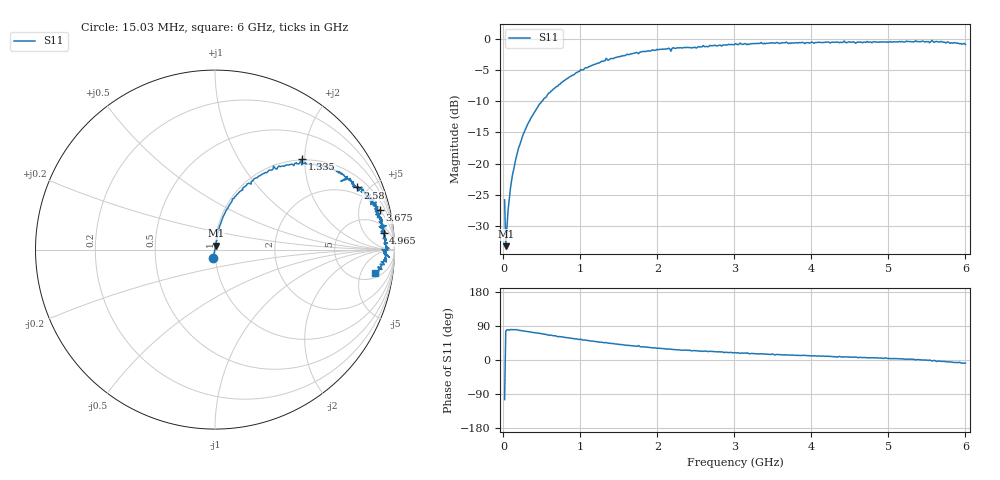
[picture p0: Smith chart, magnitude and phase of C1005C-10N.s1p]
!	Network	Analyzer	HP8753E.07.74:	Oct	30	2002	Serial	No.	JP38451487
!	Hewlett-Packard
!	7	Sep	2009	8:37:45
!	Frequency	S11
#	HZ	S	RI	R	50
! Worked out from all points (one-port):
!   400 points, 15.03 MHz to 6 GHz, reference 50 ohm
!   lowest |S11| = -33.3 dB at 30.03 MHz (marker M1), VSWR 1.04, Z = 50.5 + j2.13 ohm
!   |S11| at or under -10 dB: start of sweep to 500.2 MHz
!   S11 on the Smith chart (normalised r, x): 15.03 MHz: 0.97, -0.10; 1.335 GHz: 0.98, +1.94; 2.58 GHz: 1.55, +4.26; 3.675 GHz: 1.95, +8.01; 4.965 GHz: 9, +15; 6 GHz: 7, -9
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1.502992e7  -0.0128 -0.0495
3.002985e7  0.00513 0.0211
6.00297e7  0.0074 0.0415
1.050295e8  0.0124 0.0716
1.95029e8  0.0254 0.13
2.550287e8  0.0389 0.166
4.650277e8  0.0977 0.283
7.650262e8  0.218 0.395
1.335023e9  0.485 0.505
1.515022e9  0.545 0.471
1.99502e9  0.71 0.422
2.145019e9  0.737 0.408
2.175019e9  0.701 0.381
2.205019e9  0.754 0.396
2.265019e9  0.758 0.387
2.580017e9  0.793 0.346
3.015015e9  0.866 0.304
3.675012e9  0.919 0.22
3.765011e9  0.903 0.21
4.515007e9  0.933 0.126
4.965005e9  0.939 0.0908
5.265004e9  0.954 0.0331
5.535002e9  0.931 0.00107
5.565002e9  0.972 -0.0434
5.595002e9  0.94 -0.0179
5.625002e9  0.954 -0.0695
5.655002e9  0.947 -0.0436
6e9  0.894 -0.13
